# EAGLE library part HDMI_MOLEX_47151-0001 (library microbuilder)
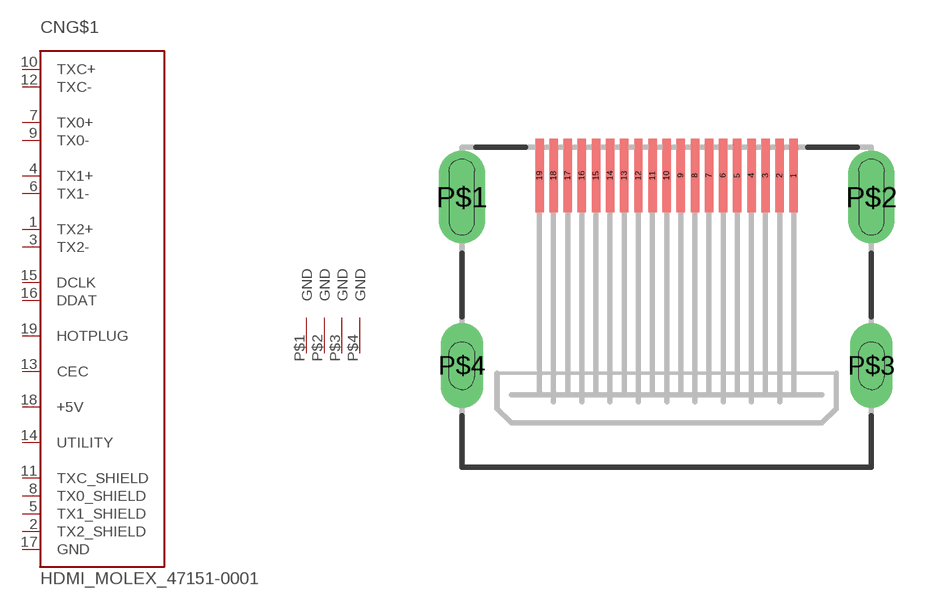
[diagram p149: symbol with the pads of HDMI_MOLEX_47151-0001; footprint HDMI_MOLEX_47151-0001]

Designator prefix CN; gates G$1=HDMI_CONN SHELL=HDMI_SHELL

## HDMI_MOLEX_47151-0001  [HDMI_MOLEX_47151-0001]
1  G$1:TX2+
2  G$1:TX2_SHIELD  pwr
3  G$1:TX2-
4  G$1:TX1+
5  G$1:TX1_SHIELD  pwr
6  G$1:TX1-
7  G$1:TX0+
8  G$1:TX0_SHIELD  pwr
9  G$1:TX0-
10  G$1:TXC+
11  G$1:TXC_SHIELD  pwr
12  G$1:TXC-
13  G$1:CEC
14  G$1:UTILITY
15  G$1:DCLK
16  G$1:DDAT
17  G$1:GND  pwr
18  G$1:+5V  pwr
19  G$1:HOTPLUG
P$1  SHELL:GND  pwr
P$2  SHELL:GND  pwr
P$3  SHELL:GND  pwr
P$4  SHELL:GND  pwr

## Footprint HDMI_MOLEX_47151-0001 (pad centres in mm)
smd 0.3 x 2.6: 1 4.5,0; 2 4,0; 3 3.5,0; 4 3,0; 5 2.5,0; 6 2,0; 7 1.5,0; 8 1,0; 9 0.5,0; 10 0,0; 11 -0.5,0; 12 -1,0; 13 -1.5,0; 14 -2,0; 15 -2.5,0; 16 -3,0; 17 -3.5,0; 18 -4,0; 19 -4.5,0
drill 0.9 pad 1.65 long: P$1 -7.25,-0.76; P$2 7.25,-0.76
drill 0.9 pad 1.5 long: P$3 7.25,-6.72; P$4 -7.25,-6.72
